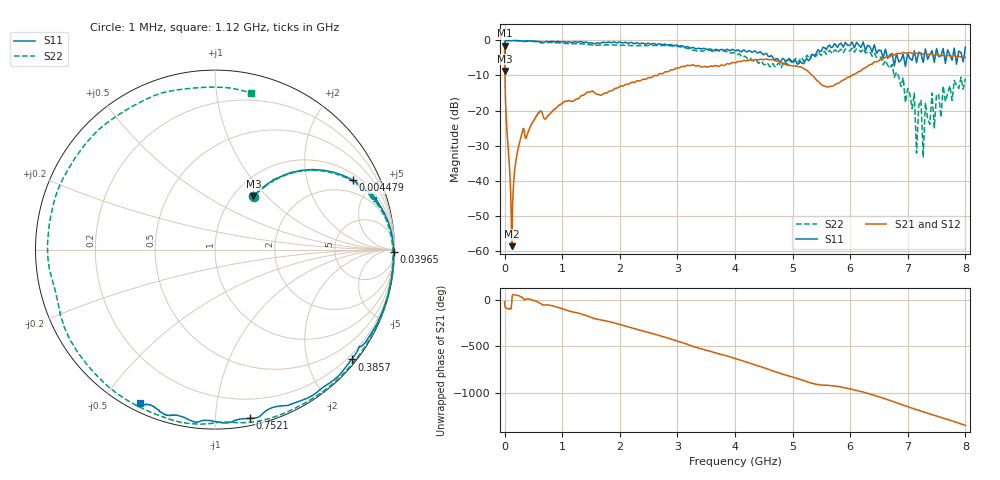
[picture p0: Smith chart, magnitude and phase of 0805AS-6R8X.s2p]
!s-Parameter Generated by FASTRON Sdn. Bhd.
!FASTRON P/N : 0805AS-6R8X
!Keysight Technologies: E4991B_MY54100416_A.01.15
!Date: Mon Jun 15 12:59:54 2026
!Version  :Rev01  Mon Jun 15 12:59:54 2026
!Data & Calibration Information:
!Freq  S11  S21  S12  S22
!PortZ  Port1:50+j0  Port2:50+j0
!When reading reference impedance value at option line is always used.
! Remarks : This data is being provided solely for informational purposes.
!PortZ  Port1:50+j0  Port2:50+j0
!Above PortZ is port z conversion or system Z0 setting when saving the data.
! "!When reading, reference impedance value at option line is always used."
# Hz S dB R 50
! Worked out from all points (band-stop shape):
!   1601 points, 1 MHz to 8 GHz, reference 50 ohm
!   highest |S21| = -1.51 dB at 1.013 MHz (marker M1); lowest = -58.6 dB at 125.5 MHz (marker M2)
!   |S21| within 3 dB of the highest: start of sweep to 3.009 MHz; 6.702 GHz to 7.829 GHz (1.126 GHz wide, 15.5 % of centre)
!   lowest |S11| = -8.7 dB at 1 MHz (marker M3), VSWR 2.15, Z = 61.5 + j42 ohm
!   |S11| at or under -10 dB: nowhere
!   |S22| runs from -33.2 to 0.0 dB; largest |S21 - S12| = 0.012
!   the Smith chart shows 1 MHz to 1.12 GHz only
!   S11 on the Smith chart (normalised r, x): 1 MHz: 1.23, +0.84; 4.479 MHz: 1.28, +3.81; 39.65 MHz: open; 385.7 MHz: 0.11, -2.84; 752.1 MHz: 0.05, -1.23; 1.12 GHz: 0.03, -0.62
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1000000  -8.74 54.1  -1.51 -20.9  -1.50 -20.8  -8.74 53.9
1013202  -8.72 53.9  -1.51 -21.0  -1.52 -20.9  -8.71 53.6
4479405  -1.31 26.7  -6.79 -59.9  -6.77 -59.8  -1.32 26.1
2.00676e7  -0.09 4.6  -18.80 -84.9  -18.70 -84.8  -0.10 1.7
3.965227e7  -0.04 -0.8  -25.20 -91.1  -25.20 -91.0  -0.06 -6.4
8.994653e7  -0.03 -8.1  -37.50 -98.4  -37.50 -99.3  -0.03 -21.0
1.255243e8  -0.03 -12.7  -58.60 -11.0  -58.50 -14.2  -0.04 -30.0
3.856923e8  -0.21 -38.8  -27.30 9.5  -27.20 9.4  -0.18 -98.0
4.006501e8  -0.19 -41.2  -26.50 10.2  -26.50 10.1  -0.17 -101.0
7.521334e8  -0.35 -78.3  -21.50 -54.9  -21.50 -55.1  -0.60 170.0
1.120185e9  -0.43 -116.0  -17.20 -120.0  -17.20 -120.0  -0.97 76.9
1.7949e9  -0.48 -178.0  -14.70 129.0  -14.80 129.0  -1.29 -87.0
2.146431e9  -0.84 144.0  -12.50 69.9  -12.50 69.8  -1.42 -178.0
2.516241e9  -0.97 105.0  -10.60 6.1  -10.60 6.0  -1.46 93.1
2.883048e9  -1.16 64.1  -8.45 -58.9  -8.45 -58.9  -1.57 4.6
3.223742e9  -2.20 31.0  -7.19 -128.0  -7.18 -128.0  -2.48 -84.0
3.933151e9  -2.77 -39.4  -6.52 106.0  -6.49 105.0  -3.63 101.0
4.632554e9  -4.30 -103.0  -5.45 -35.2  -5.48 -35.7  -7.01 -95.7
5.248374e9  -5.20 -118.0  -8.51 -157.0  -8.55 -157.0  -4.21 161.0
5.840928e9  -0.81 172.0  -11.60 147.0  -11.60 146.0  -2.49 5.7
7.151793e9  -6.37 64.7  -3.70 -96.9  -3.71 -97.6  -32.10 55.0
8e9  -1.88 -16.9  -4.85 94.8  -4.72 94.8  -10.90 -87.3
